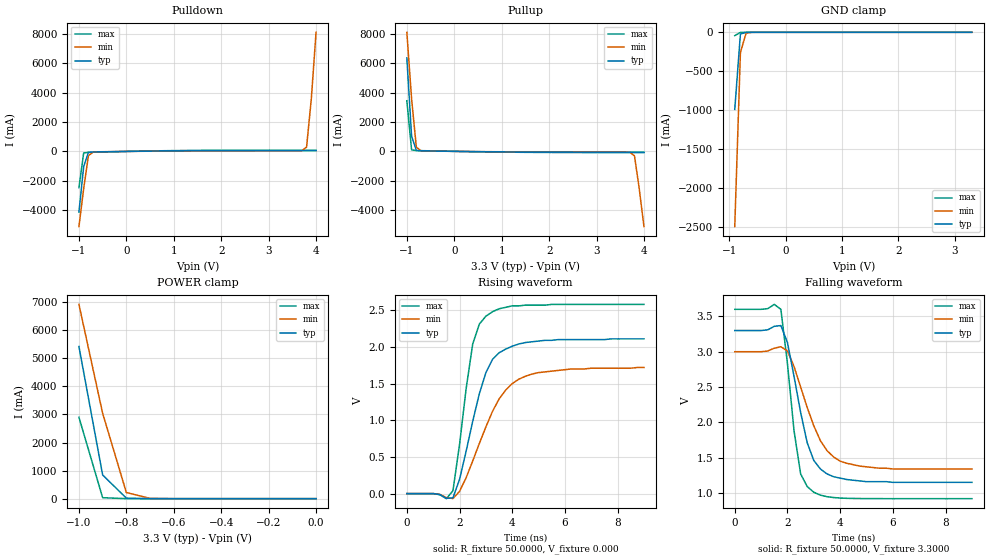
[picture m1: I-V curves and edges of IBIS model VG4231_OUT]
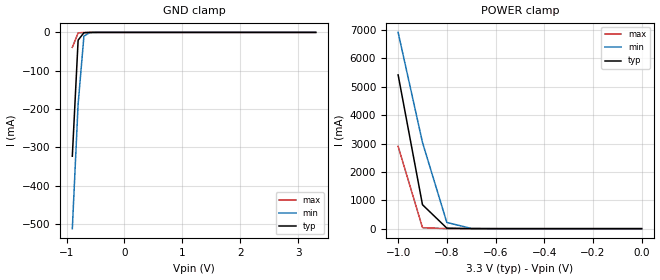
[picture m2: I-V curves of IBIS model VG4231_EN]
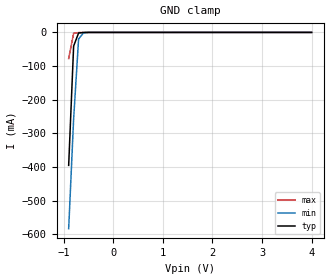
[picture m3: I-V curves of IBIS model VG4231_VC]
[IBIS ver]   2.1
[File name]   423bcacf.ibs
[File Rev]   0.1
[Date]   November 12, 2007
[Copyright]   EPSONTOYOCOM Corp.
|   Component VG-4231CAxxC
[Component]   VG-4231CAxxC
[Manufacturer]   EPSONTOYOCOM Corp.
[Package]
| variable   typ   min   max
R_pkg   0.20   0.13   0.28
L_pkg   5.16nH   4.56nH   5.76nH
C_pkg   1.23pF   1.03pF   1.53pF
[Pin]  signal_name   model_name   R_pin   L_pin   C_pin
1   VC   VG4231_VC
2   NC   NC
3   GND   GND
4   OUT   VG4231_OUT
5   OE   VG4231_EN
6   VDD   POWER
| Models and submodels in the file (3): VG4231_OUT (3-state), VG4231_EN (Input), VG4231_VC (Input)
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|   Model VG4231_OUT
[Model]   VG4231_OUT
Model_type   3-state
Polarity   Non-Inverting
Enable   Active-High
C_comp   2.2010pF   2.2010pF   2.2010pF
[Temperature Range]   27.0000   85.0000   -40.0000
[Voltage Range]   3.3000V   3.0000V   3.6000V
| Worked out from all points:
|   slope of the pulldown table from 0 to 0.495 V, typ, clamps not added: 21.3 ohm
|   slope of the pullup table from 0 to 0.495 V, typ, clamps not added: 23.1 ohm
|   GND clamp passes 1 mA (typ) near -0.70 V on its own axis
|   POWER clamp passes 1 mA (typ) near -0.70 V on its own axis
|   rising waveform, R_fixture 50.0000, V_fixture 0.000: 20-80 % time 904ps typ, 1.29ns min, 583ps max; typ from 0 V to 2.11 V
|   falling waveform, R_fixture 50.0000, V_fixture 3.3000: 20-80 % time 745ps typ, 1.02ns min, 500ps max; typ from 3.3 V to 1.15 V
[Pulldown]
| voltage   I(typ)   I(min)   I(max)
-1V       -4.13A     -5.12A     -2.47A
-900mV    -1.03A     -2.53A     -108mA
-800mV    -64.8mA    -292mA     -60.4mA
-700mV    -38.7mA    -39.1mA    -53mA
1.2V      44.2mA     31.8mA     63.8mA
3.6V      55.6mA     40mA       79.6mA
3.7V      55.7mA     50.1mA     79.7mA
3.8V      55.8mA     294mA      79.8mA
3.9V      55.9mA     3.58A      79.8mA
4V        56.6mA     8.12A      79.9mA
[Pullup]
| voltage   I(typ)   I(min)   I(max)
-1V       6.37A      8.12A      3.45A
-900mV    1.03A      3.58A      102mA
-800mV    63.1mA     287mA      55.6mA
-700mV    37.2mA     39.9mA     48.2mA
-600mV    31.3mA     25.8mA     41.2mA
1.3V      -44.6mA    -34.7mA    -60.7mA
3.7V      -60.9mA    -56.8mA    -83.7mA
3.8V      -61.1mA    -307mA     -83.9mA
3.9V      -61.4mA    -2.54A     -84.1mA
4V        -62.4mA    -5.13A     -84.3mA
[GND_clamp]
| voltage   I(typ)   I(min)   I(max)
-900mV    -988mA     -2.49A     -42.8mA
-800mV    -22.3mA    -261mA     -1.3mA
-700mV    -968uA     -10.8mA    -315uA
-500mV    -14.7uA    -62uA      -1.68uA
3.3V      74.5pA     1.33uA     63.6pA
[POWER_clamp]
| voltage   I(typ)   I(min)   I(max)
-1V       5.42A      6.92A      2.9A
-900mV    844mA      3.04A      34.8mA
-800mV    18.4mA     218mA      463uA
-700mV    660uA      9.21mA     37.4uA
-600mV    72.5uA     610uA      3.68uA
-500mV    9.26uA     82.1uA     222nA
-400mV    866nA      11.7uA     6.61nA
-300mV    50.9nA     1.33uA     219pA
-200mV    2.14nA     106nA      91.4pA
-100mV    142pA      6.18nA     84.4pA
0V        74.5pA     170pA      79.2pA
[Ramp]
| variable   typ   min   max
dV/dt_r   1.27/0.888n   1.03/1.28n   1.55/0.567n
dV/dt_f   1.29/0.716n   1.00/1.01n   1.61/0.457n
R_load = 50.0000
[Rising Waveform]
R_fixture = 50.0000
V_fixture = 0.000
V_fixture_min = 0.000
V_fixture_max = 0.000
| time   V(typ)   V(min)   V(max)
0s        1.25nV     8.65nV     996pV
1.5ns     -65.6mV    -55.6mV    -69.4mV
1.75ns    -57.6mV    -68mV      39.6mV
2ns       193mV      29.5mV     669mV
2.5ns     986mV      445mV      2.04V
2.75ns    1.36V      682mV      2.31V
3ns       1.65V      909mV      2.42V
3.75ns    1.97V      1.41V      2.54V
4.5ns     2.06V      1.6V       2.57V
9ns       2.11V      1.72V      2.58V
[Falling Waveform]
R_fixture = 50.0000
V_fixture = 3.3000
V_fixture_min = 3.0000
V_fixture_max = 3.6000
| time   V(typ)   V(min)   V(max)
0s        3.3V       3V         3.6V
1.75ns    3.37V      3.07V      3.6V
2ns       3.13V      3.01V      2.83V
2.25ns    2.65V      2.79V      1.88V
2.5ns     2.14V      2.5V       1.27V
2.75ns    1.71V      2.21V      1.09V
3ns       1.46V      1.95V      1.01V
3.5ns     1.27V      1.6V       947mV
4.25ns    1.19V      1.42V      924mV
9ns       1.15V      1.34V      919mV
|   Model VG4231_EN
[Model]   VG4231_EN
Model_type   Input
Vinl =   0.6600V
Vinh =   2.6400V
C_comp   1.4070pF   1.4070pF   1.4070pF
[Temperature Range]   27.0000   85.0000   -40.0000
[Voltage Range]   3.3000V   3.0000V   3.6000V
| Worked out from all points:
|   GND clamp passes 1 mA (typ) near -0.70 V on its own axis
|   POWER clamp passes 1 mA (typ) near -0.70 V on its own axis
[GND_clamp]
| voltage   I(typ)   I(min)   I(max)
-900mV    -323mA     -512mA     -39mA
-800mV    -20.3mA    -187mA     -1.24mA
-700mV    -916uA     -9.88mA    -313uA
-600mV    -139uA     -599uA     -39.6uA
-500mV    -16.2uA    -62uA      -3.84uA
3.3V      18.4pA     290nA      -498nA
[POWER_clamp]
| voltage   I(typ)   I(min)   I(max)
-1V       5.42A      6.92A      2.9A
-900mV    844mA      3.04A      34.8mA
-800mV    18.4mA     218mA      463uA
-700mV    660uA      9.21mA     37.4uA
-600mV    72.5uA     610uA      3.68uA
-500mV    9.26uA     82.1uA     222nA
-400mV    866nA      11.7uA     6.61nA
-300mV    50.9nA     1.33uA     219pA
-200mV    2.14nA     106nA      91.4pA
-100mV    142pA      6.18nA     84.4pA
0V        74.5pA     170pA      79.2pA
|   Model VG4231_VC
[Model]   VG4231_VC
Model_type   Input
Vinl =   0.800V
Vinh =   2.000V
C_comp   1.4070pF   1.4070pF   1.4070pF
[Temperature Range]   27.0000   85.0000   -40.0000
[Voltage Range]   3.3000V   3.0000V   3.6000V
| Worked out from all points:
|   GND clamp passes 1 mA (typ) near -0.65 V on its own axis
[GND_clamp]
| voltage   I(typ)   I(min)   I(max)
-900mV    -395mA     -583mA     -77.7mA
-800mV    -40.6mA    -257mA     -2.48mA
-700mV    -1.84mA    -19.7mA    -632uA
-600mV    -282uA     -1.2mA     -81.5uA
4V        33.3uA     28.6uA     40uA
